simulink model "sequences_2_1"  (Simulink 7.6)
settings: Solver=ode15s  StartTime=0.0  StopTime=3/60  RelTol=1e-3
InitFcn:
  | clc
  | close all
  | 
  | % Résistance et inductance de la source
  | Rg=1;
  | Lg=1e-6;
  | 
  | % Charges
  | % charge de la phase C
  | R1=2;
  | 
  | % Charge R, L de la phase B
  | R=1;
  | L=0.1;
StopFcn:
  | load phases_syst_triphase.mat
  | 
  | plot(x(1,:),x(2,:),x(1,:),x(3,:),'LineWidth',3);
  | hold on
  | 
  | plot(x(1,:),x(4,:),x(1,:),x(5,:),'LineWidth',2);
  | hold on
  | 
  | plot(x(1,:),x(6,:),x(1,:),x(7,:),'LineWidth',1);
  | title('Amplitudes et phases du système triphasé')
  | xlabel('temps')
  | grid
undefined symbols (not defined in the file or in its folder): Angle, Magnitude, Ts
libraries: powerlib x11, powerlib_extras x5

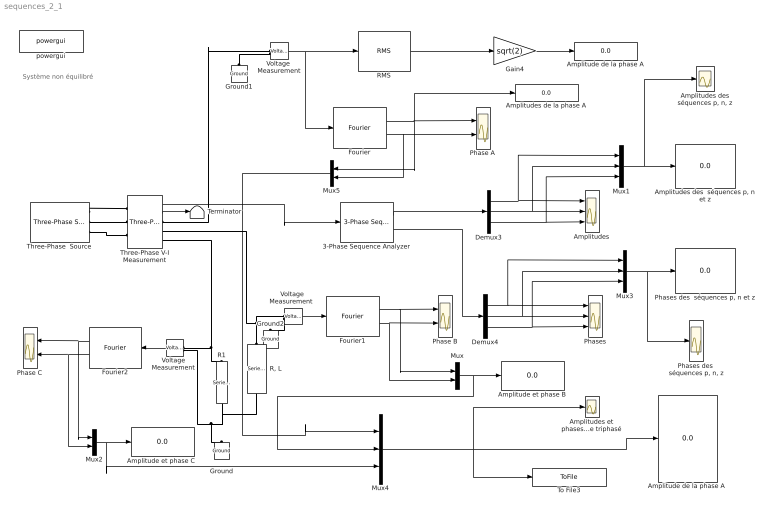
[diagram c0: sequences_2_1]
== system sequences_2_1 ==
  note: Système non équilibré
  3-Phase Sequence Analyzer : powerlib_extras/Measurements/3-Phase Sequence Analyzer  DialogController=POWERSYS.PowerSysDialog  SystemSampleTime=-1  f1=60  n=1  seq=Positive Negative Zero
  Amplitude de la phase A : Display
  "Amplitude de la phase A " : Display
  Amplitude et phase B : Display
  "Amplitude et phase C " : Display
  Amplitudes : Scope  NumInputPorts=3
  Amplitudes de la phase A : Display
  "Amplitudes des séquences p, n, z" : Scope
  "Amplitudes des  séquences p, n et z" : Display
  Amplitudes et phases  du système triphasé : Scope
  Demux3 : Demux  Outputs=3
  Demux4 : Demux  Outputs=3
  Fourier : powerlib_extras/Measurements/Fourier  DialogController=POWERSYS.PowerSysDialog  SystemSampleTime=-1  f1=60  n=1
  Fourier1 : powerlib_extras/Measurements/Fourier  DialogController=POWERSYS.PowerSysDialog  SystemSampleTime=-1  f1=60  n=1
  Fourier2 : powerlib_extras/Measurements/Fourier  DialogController=POWERSYS.PowerSysDialog  SystemSampleTime=-1  f1=60  n=1
  Gain4 : Gain  Gain=sqrt(2)
  Ground : powerlib/Elements/Ground  DialogController=POWERSYS.PowerSysDialog  PhysicalDomain=powersysdomain  SubClassName=unknown  LeftPortType=p1  RightPortType=p1  LConnTagsString=a
  Ground1 : powerlib/Elements/Ground  DialogController=POWERSYS.PowerSysDialog  PhysicalDomain=powersysdomain  SubClassName=unknown  LeftPortType=p1  RightPortType=p1  LConnTagsString=a
  Ground2 : powerlib/Elements/Ground  DialogController=POWERSYS.PowerSysDialog  PhysicalDomain=powersysdomain  SubClassName=unknown  LeftPortType=p1  RightPortType=p1  LConnTagsString=a
  Mux : Mux  Inputs=2
  Mux1 : Mux  Inputs=3
  Mux2 : Mux  Inputs=2
  Mux3 : Mux  Inputs=3
  Mux4 : Mux  Inputs=3
  Mux5 : Mux  Inputs=2
  "Phase A " : Scope  NumInputPorts=2
  Phase B : Scope  NumInputPorts=2
  Phase C : Scope  NumInputPorts=2
  Phases : Scope  NumInputPorts=3
  "Phases des  séquences p, n et z" : Display
  "Phases des  séquences p, n, z" : Scope
  "R, L" : powerlib/Elements/Series RLC Branch  DialogController=POWERSYS.PowerSysDialog  PhysicalDomain=powersysdomain  SubClassName=unknown  LeftPortType=p1  RightPortType=p1  LConnTagsString=__new0  RConnTagsString=__new0  BranchType=RL  Resistance=R  Inductance=L  SetiL0=off  InitialCurrent=0  Capacitance=1e-3  Setx0=off  InitialVoltage=0  Measurements=None
  R1 : powerlib/Elements/Series RLC Branch  DialogController=POWERSYS.PowerSysDialog  PhysicalDomain=powersysdomain  SubClassName=unknown  LeftPortType=p1  RightPortType=p1  LConnTagsString=__new0  RConnTagsString=__new0  BranchType=R  Resistance=R1  Inductance=1e-3  SetiL0=off  InitialCurrent=0  Capacitance=1e-6  Setx0=off  InitialVoltage=0  Measurements=None
  RMS : powerlib_extras/Measurements/RMS  DialogController=POWERSYS.PowerSysDialog  SystemSampleTime=-1  f1=60
  Terminator : Terminator
  Three-Phase V-I Measurement : powerlib/Measurements/Three-Phase V-I Measurement  DialogController=POWERSYS.PowerSysDialog  SystemSampleTime=-1  VoltageMeasurement=phase-to-ground  SetLabelV=off  LabelV=Vabc  Vpu=off  VpuLL=off  CurrentMeasurement=yes  SetLabelI=off  LabelI=Iabc  Ipu=off  Pbase=100e6  Vbase=500e3  OutputType=Magnitude-Angle  PhasorSimulation=off  PSBequivalent=0
  Three-Phase  Source : powerlib/Electrical Sources/Three-Phase Source  DialogController=POWERSYS.PowerSysDialog  SystemSampleTime=-1  Voltage=220*sqrt(3)/sqrt(2)  PhaseAngle=0  Frequency=60  InternalConnection=Yg  SpecifyImpedance=off  Resistance=Rg  Inductance=Lg  ShortCircuitLevel=100e6  BaseVoltage=25e3  XRratio=1e-12
  To File3 : ToFile  Filename=phases_syst_triphase  MatrixName=x
  Voltage  Measurement : powerlib/Measurements/Voltage Measurement  DialogController=POWERSYS.PowerSysDialog  SystemSampleTime=-1  PhasorSimulation=off  OutputType=Complex  PSBequivalent=0
  "Voltage  Measurement " : powerlib/Measurements/Voltage Measurement  DialogController=POWERSYS.PowerSysDialog  SystemSampleTime=-1  PhasorSimulation=off  OutputType=Complex  PSBequivalent=0
  "Voltage  Measurement  " : powerlib/Measurements/Voltage Measurement  DialogController=POWERSYS.PowerSysDialog  SystemSampleTime=-1  PhasorSimulation=off  OutputType=Complex  PSBequivalent=0
  powergui : powerlib/powergui  Priority=1  SystemSampleTime=-1  SimulationMode=Continuous  SampleTime=Ts  frequency=60  SPID=off  DisableSnubberDevices=off  DisableRonSwitches=off  DisableVfSwitches=off  SwTol=0  Interpol=off  frequencyindice=60  echomessages=off  HookPort=off  DisplayEquations=off  FunctionMessages=off  EnableUseOfTLC=off  x0status=blocks  RestoreLinks=warning  ResistiveCurrentMeasurement=off  Ylog=off  Xlog=on  ShowGrid=off  save=off  variable=ZData  ZoomFFT=off  StartTime=0.0  cycles=1  DisplayStyle=1  FreqAxis=off  MaxFrequency=1000  frequencyindicesteady=1  display=off  methode=off
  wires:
  3-Phase Sequence Analyzer/1 -> Demux3/1
  Demux3/1 -> Mux1/1, Amplitudes/1
  Demux4/1 -> Mux3/1, Phases/1
  Demux4/2 -> Mux3/2, Phases/2
  Demux4/3 -> Mux3/3, Phases/3
  Mux3/1 -> "Phases des  séquences p, n et z"/1, "Phases des  séquences p, n, z"/1
  3-Phase Sequence Analyzer/2 -> Demux4/1
  Demux3/2 -> Amplitudes/2, Mux1/2
  Demux3/3 -> Amplitudes/3, Mux1/3
  Mux1/1 -> "Amplitudes des  séquences p, n et z"/1, "Amplitudes des séquences p, n, z"/1
  Voltage  Measurement/1 -> RMS/1, Fourier/1
  RMS/1 -> Gain4/1
  Gain4/1 -> Amplitude de la phase A/1
  Fourier/1 -> "Phase A "/1, Amplitudes de la phase A/1, Mux5/1
  Fourier/2 -> "Phase A "/2, Mux5/2
  "Voltage  Measurement "/1 -> Fourier2/1
  Fourier2/1 -> Phase C/1, Mux2/1
  Fourier2/2 -> Phase C/2, Mux2/2
  Fourier1/1 -> Phase B/1, Mux/1
  Fourier1/2 -> Phase B/2, Mux/2
  "Voltage  Measurement  "/1 -> Fourier1/1
  Mux/1 -> Amplitude et phase B/1, Mux4/2
  Mux2/1 -> "Amplitude et phase C "/1, Mux4/3
  Three-Phase V-I Measurement/1 -> 3-Phase Sequence Analyzer/1
  Mux4/1 -> Amplitudes et phases  du système triphasé/1, "Amplitude de la phase A "/1, To File3/1
  Three-Phase V-I Measurement/2 -> Terminator/1
  Mux5/1 -> Mux4/1
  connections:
  "Voltage  Measurement "/LConn1 -- R1/RConn1 -- Three-Phase V-I Measurement/RConn3
  "R, L"/LConn1 -- "Voltage  Measurement  "/LConn1 -- Three-Phase V-I Measurement/RConn2
  "Voltage  Measurement "/LConn2 -- R1/LConn1 -- Ground/LConn1 -- "R, L"/RConn1
  Ground1/LConn1 -- Voltage  Measurement/LConn2
  "Voltage  Measurement  "/LConn2 -- Ground2/LConn1
  Three-Phase  Source/RConn1 -- Three-Phase V-I Measurement/LConn1
  Three-Phase  Source/RConn2 -- Three-Phase V-I Measurement/LConn2
  Three-Phase  Source/RConn3 -- Three-Phase V-I Measurement/LConn3
  Three-Phase V-I Measurement/RConn1 -- Voltage  Measurement/LConn1
